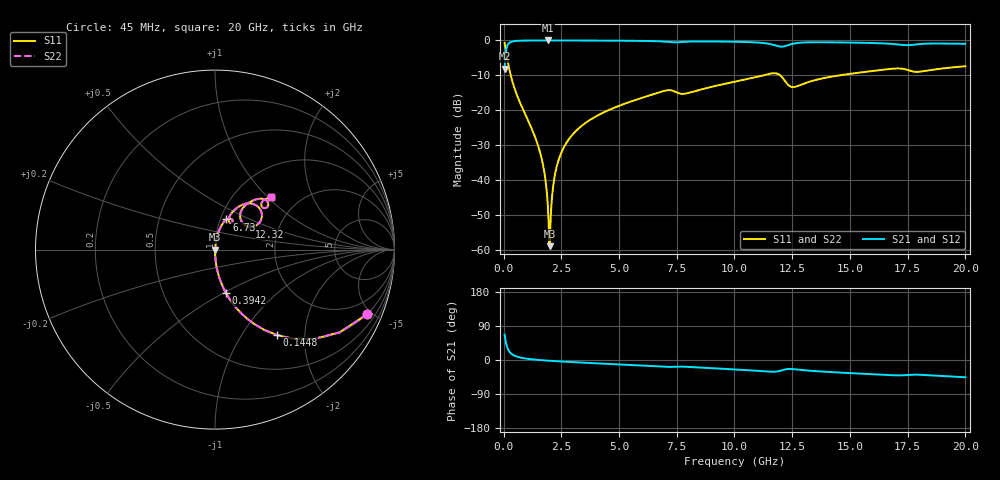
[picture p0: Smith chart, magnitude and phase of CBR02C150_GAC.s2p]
! S-parameter model data by Modelithics Inc.  support@modelithics.com 813-866-6335  Tampa FL USA
! S-Parameter data specifications:
! Substrate: 20-mil Rogers 4350B, substrate thickness, H=0.508mm, Dielectric constant, Er=3.75
! PCB Mounting Pad Footprint: Pad width, PadW=0.32mm , Pad length, PadL=0.37mm , Pad gap, PadG (edge-to-edge)=0.19mm , Reference planes=0.93mm apart
#  GHz  S  MA  R 50
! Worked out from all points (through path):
!   801 points, 45 MHz to 20 GHz, reference 50 ohm
!   highest |S21| = -0.01 dB at 1.916 GHz (marker M1); lowest = -8.1 dB at 45 MHz (marker M2)
!   group delay of S21, straight-line fit = 7.14 ps
!   lowest |S11| = -59.0 dB at 1.991 GHz (marker M3), VSWR 1.00, Z = 50.1 - j0.00805 ohm
!   |S11| at or under -10 dB: 309.3 MHz to 11.25 GHz (10.94 GHz wide, 189 % of centre); 11.98 GHz to 14.57 GHz (2.593 GHz wide, 19.5 % of centre)
!   |S22| runs from -59.0 to -0.7 dB; largest |S21 - S12| = 0
!   S11 on the Smith chart (normalised r, x): 45 MHz: 1.00, -4.68; 144.8 MHz: 1.00, -1.45; 394.2 MHz: 1.00, -0.51; 6.73 GHz: 1.07, +0.37; 12.32 GHz: 1.42, +0.38; 20 GHz: 1.46, +1.04
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0.045  0.9199 -23.1  0.392 66.9  0.392 66.9  0.9199 -23.1
0.144775  0.5872 -54.1  0.809 35.8  0.809 35.8  0.5872 -54.1
0.24455  0.3914 -67.1  0.9197 22.8  0.9197 22.8  0.3914 -67.1
0.394213  0.2492 -75.8  0.9678 14.0  0.9678 14.0  0.2492 -75.8
1.566569  0.02576 -87.9  0.9986 -0.1  0.9986 -0.1  0.02576 -87.9
1.791063  0.01135 -85.8  0.9988 -1.2  0.9988 -1.2  0.01135 -85.8
1.915781  0.004264 -76.7  0.9989 -1.7  0.9989 -1.7  0.004264 -76.7
1.990612  0.00112 -4.1  0.9988 -2.0  0.9988 -2.0  0.00112 -4.1
2.065444  0.004052 71.4  0.9988 -2.3  0.9988 -2.3  0.004052 71.4
2.215106  0.01143 81.2  0.9987 -2.9  0.9987 -2.9  0.01143 81.2
2.414656  0.02072 83.0  0.9985 -3.6  0.9985 -3.6  0.02072 83.0
2.788813  0.03669 83.0  0.998 -4.9  0.998 -4.9  0.03669 83.0
3.387462  0.0597 81.8  0.9967 -6.9  0.9967 -6.9  0.0597 81.8
6.704981  0.1786 69.4  0.9728 -17.1  0.9728 -17.1  0.1786 69.4
6.729925  0.1797 69.1  0.972 -17.2  0.972 -17.2  0.1797 69.1
7.852394  0.1721 62.6  0.9563 -17.7  0.9563 -17.7  0.1721 62.6
10.0225  0.2554 63.0  0.9574 -25.0  0.9574 -25.0  0.2554 63.0
11.74362  0.3382 43.4  0.8539 -30.9  0.8539 -30.9  0.3382 43.4
12.31733  0.232 33.5  0.855 -23.7  0.855 -23.7  0.232 33.5
13.36496  0.2628 56.0  0.9408 -28.7  0.9408 -28.7  0.2628 56.0
16.68248  0.3883 46.8  0.898 -39.7  0.898 -39.7  0.3883 46.8
20  0.4263 43.1  0.8947 -45.6  0.8947 -45.6  0.4263 43.1
